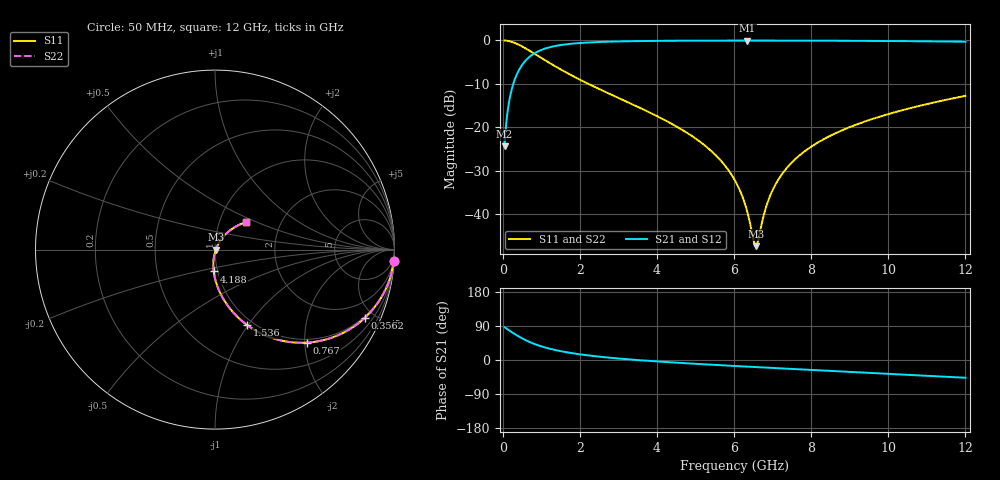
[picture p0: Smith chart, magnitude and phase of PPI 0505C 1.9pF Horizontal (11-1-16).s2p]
# GHz S MA R 50
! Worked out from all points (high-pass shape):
!   1601 points, 50 MHz to 12 GHz, reference 50 ohm
!   highest |S21| = -0.04 dB at 6.346 GHz (marker M1); lowest = -24.4 dB at 50 MHz (marker M2)
!   |S21| within 3 dB of the highest: 811.5 MHz to end of sweep
!   lowest |S11| = -47.3 dB at 6.57 GHz (marker M3), VSWR 1.01, Z = 50.4 - j0.13 ohm
!   |S11| at or under -10 dB: 2.223 GHz to end of sweep
!   |S22| runs from -47.3 to 0.0 dB; largest |S21 - S12| = 0
!   S11 on the Smith chart (normalised r, x): 50 MHz: 1, -32; 356.2 MHz: 0.93, -4.44; 767 MHz: 0.93, -2.04; 1.536 GHz: 0.93, -0.98; 4.188 GHz: 0.96, -0.24; 12 GHz: 1.34, +0.43
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0.05  0.9982 -3.6  0.06039 86.4  0.06039 86.4  0.9982 -3.6
0.1844375  0.9759 -13.1  0.2179 76.9  0.2179 76.9  0.9759 -13.1
0.3562187  0.9177 -24.4  0.3965 65.6  0.3965 65.6  0.9177 -24.4
0.767  0.7282 -45.4  0.6839 44.5  0.6839 44.5  0.7282 -45.4
1.1255  0.5811 -57.5  0.812 32.3  0.812 32.3  0.5811 -57.5
1.536281  0.455 -67.1  0.8882 22.6  0.8882 22.6  0.455 -67.1
2.044156  0.3461 -75.2  0.9356 14.4  0.9356 14.4  0.3461 -75.2
4.038312  0.1321 -92.5  0.9876 -4.0  0.9876 -4.0  0.1321 -92.5
4.187688  0.1222 -93.4  0.9888 -5.0  0.9888 -5.0  0.1222 -93.4
5.337875  0.05702 -98.1  0.9942 -12.0  0.9942 -12.0  0.05702 -98.1
6.025  0.02444 -96.2  0.9952 -15.8  0.9952 -15.8  0.02444 -96.2
6.346156  0.01057 -84.0  0.9953 -17.6  0.9953 -17.6  0.01057 -84.0
6.510469  0.004951 -48.7  0.9953 -18.4  0.9953 -18.4  0.004951 -48.7
6.570219  0.004298 -17.5  0.9953 -18.7  0.9953 -18.7  0.004298 -17.5
6.629969  0.005081 12.7  0.9953 -19.1  0.9953 -19.1  0.005081 12.7
6.8615  0.01332 50.4  0.9951 -20.3  0.9951 -20.3  0.01332 50.4
7.1005  0.02307 57.3  0.9948 -21.5  0.9948 -21.5  0.02307 57.3
7.488875  0.03902 59.7  0.9941 -23.5  0.9941 -23.5  0.03902 59.7
8.019156  0.06063 59.2  0.9928 -26.2  0.9928 -26.2  0.06063 59.2
8.870594  0.09523 56.3  0.9897 -30.6  0.9897 -30.6  0.09523 56.3
10.01331  0.1425 51.3  0.9835 -36.4  0.9835 -36.4  0.1425 51.3
12  0.2303 41.5  0.9657 -46.9  0.9657 -46.9  0.2303 41.5
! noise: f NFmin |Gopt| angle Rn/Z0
0.05  0.000879  0.9511  1.675  0.004033
1.372  0.005654  0.76  5.222  0.004763
2.701  0.008924  0.7085  8.669  0.00599
4.031  0.01182  0.6779  12.16  0.007013
5.36  0.01456  0.6575  15.62  0.007967
6.682  0.01722  0.6437  19.02  0.00891
8.012  0.01992  0.6348  22.38  0.009899
9.341  0.0227  0.6298  25.67  0.01097
10.67  0.0256  0.6283  28.9  0.01215
12  0.02869  0.6298  32.06  0.01349
